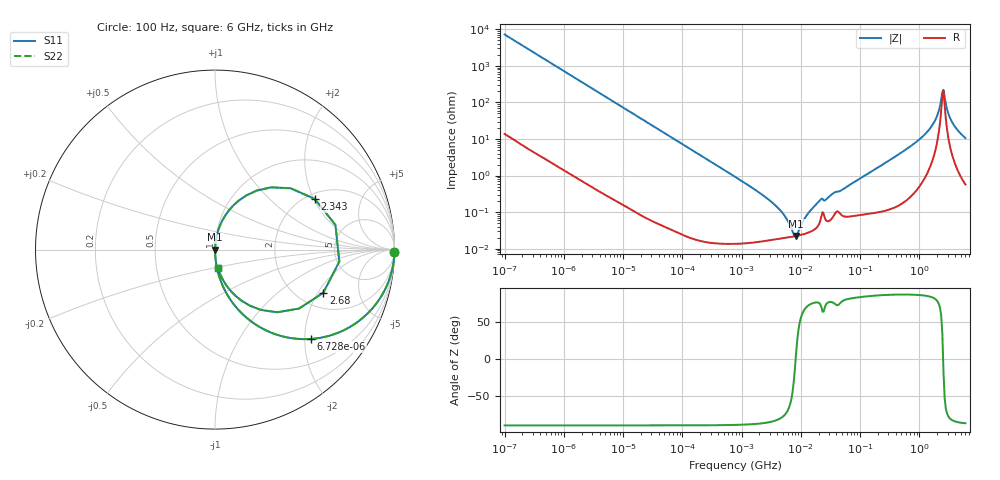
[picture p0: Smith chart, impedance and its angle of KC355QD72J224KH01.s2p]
!Murata Part Number: KC355QD72J224KH01
!These Parameters are Measured in Series Mode Connection
!Data Generated on Mar 13, 2026
!  o--ll--o
!Port1  Port2
!  o------o
!Operation Temp=25[degC], DC Bias Voltage=0[V]
!Freq. Start=100[Hz] Stop=6[GHz] 401[Steps]
# Hz S RI R 50
!Freq.(Hz) S11(Real) S11(Imag) S21(Real) S21(Imag) S12(Real) S12(Imag) S22(Real) S22(Imag)
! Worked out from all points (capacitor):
!   401 points, 100 Hz to 6 GHz, reference 50 ohm
!   read as one part in series: C = 221 nF near 109 Hz
!   lowest |Z| = 22.4 mohm at 8.312 MHz (marker M1)
!   series resonance near 8.181 MHz, so ESL is about 1.7 nH
!   S11 on the Smith chart (normalised r, x): 100 Hz: open; 6.728 kHz: 1.00, -2.15; 2.343 GHz: 2.21, +2.04; 2.68 GHz: 2.68, -2.23; 6 GHz: 1.01, -0.21
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100  0.9998 -0.0139  0.000219 0.0139  0.000219 0.0139  0.9998 -0.0139
600  0.993 -0.0825  0.00701 0.0825  0.00701 0.0825  0.993 -0.0825
2008  0.9279 -0.2577  0.0721 0.2577  0.0721 0.2577  0.9279 -0.2577
6728  0.5365 -0.4976  0.4635 0.4976  0.4635 0.4976  0.5365 -0.4976
15752  0.1753 -0.3791  0.8247 0.3791  0.8247 0.3791  0.1753 -0.3791
40335  0.0318 -0.1741  0.9682 0.1741  0.9682 0.1741  0.0318 -0.1741
774597  0.000222 -0.00928  0.9998 0.00928  0.9998 0.00928  0.000222 -0.00928
3712478  0.000182 -0.00153  0.9998 0.00153  0.9998 0.00153  0.000182 -0.00153
5311619  0.000197 -0.000776  0.9998 0.000776  0.9998 0.000776  0.000197 -0.000776
7599586  0.000216 -0.000128  0.9998 0.000128  0.9998 0.000128  0.000216 -0.000128
8311524  0.000223 2.8e-05  0.9998 -2.8e-05  0.9998 -2.8e-05  0.000223 2.8e-05
1.555665e7  0.000309 0.00121  0.9997 -0.00121  0.9997 -0.00121  0.000309 0.00121
2.128304e7  0.000579 0.00209  0.9994 -0.00209  0.9994 -0.00209  0.000579 0.00209
3.124326e8  0.00185 0.026  0.9981 -0.026  0.9981 -0.026  0.00185 0.026
8.749838e8  0.0103 0.0803  0.9897 -0.0803  0.9897 -0.0803  0.0103 0.0803
1.565993e9  0.0579 0.1912  0.9421 -0.1912  0.9421 -0.1912  0.0579 0.1912
1.95892e9  0.1749 0.302  0.8251 -0.302  0.8251 -0.302  0.1749 0.302
2.34314e9  0.5558 0.282  0.4442 -0.282  0.4442 -0.282  0.5558 0.282
2.679998e9  0.603 -0.2406  0.397 0.2406  0.397 0.2406  0.603 -0.2406
2.931063e9  0.3473 -0.3491  0.6527 0.3491  0.6527 0.3491  0.3473 -0.3491
3.505958e9  0.1158 -0.2589  0.8842 0.2589  0.8842 0.2589  0.1158 -0.2589
6e9  0.0166 -0.1034  0.9834 0.1034  0.9834 0.1034  0.0166 -0.1034
